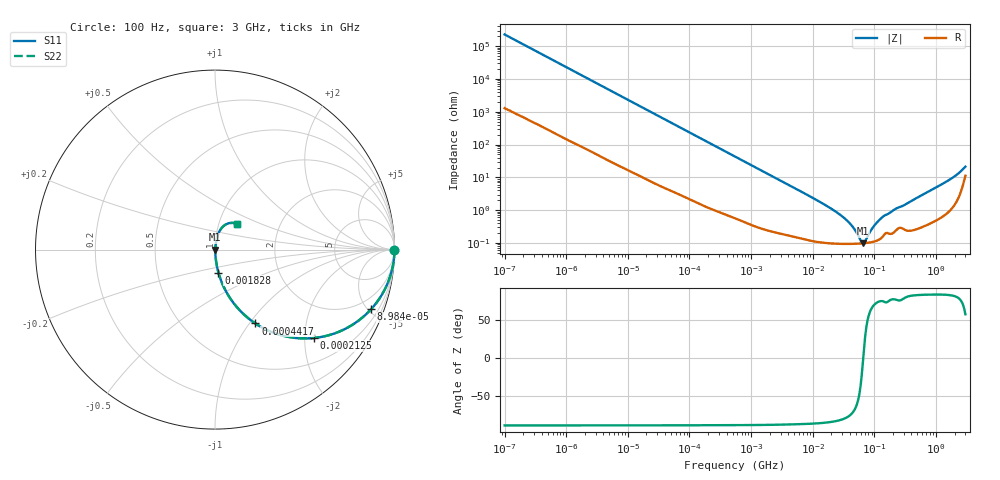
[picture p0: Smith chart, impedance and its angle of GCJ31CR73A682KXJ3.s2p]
!Murata Part Number: GCJ31CR73A682KXJ3
!These Parameters are Measured in Series Mode Connection
!Data Generated on Mar 13, 2026
!  o--ll--o
!Port1  Port2
!  o------o
!Operation Temp=25[degC], DC Bias Voltage=0[V]
!Freq. Start=100[Hz] Stop=3[GHz] 401[Steps]
# Hz S RI R 50
!Freq.(Hz) S11(Real) S11(Imag) S21(Real) S21(Imag) S12(Real) S12(Imag) S22(Real) S22(Imag)
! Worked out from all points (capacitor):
!   401 points, 100 Hz to 3 GHz, reference 50 ohm
!   read as one part in series: C = 7 nF near 109 Hz
!   lowest |Z| = 98.1 mohm at 65.08 MHz (marker M1)
!   series resonance near 65.93 MHz, so ESL is about 830 pH
!   S11 on the Smith chart (normalised r, x): 100 Hz: open; 89.84 kHz: 1.05, -5.21; 212.5 kHz: 1.02, -2.21; 441.7 kHz: 1.01, -1.07; 1.828 MHz: 1.00, -0.26; 3 GHz: 1.22, +0.36
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100  1 -0.00044  2.7e-06 0.00044  2.7e-06 0.00044  1 -0.00044
1788  0.9999 -0.00778  0.000112 0.00778  0.000112 0.00778  0.9999 -0.00778
10443  0.9976 -0.045  0.00236 0.045  0.00236 0.045  0.9976 -0.045
31977  0.9804 -0.1346  0.0196 0.1346  0.0196 0.1346  0.9804 -0.1346
89839  0.8692 -0.3327  0.1308 0.3327  0.1308 0.3327  0.8692 -0.3327
212480  0.5496 -0.4924  0.4504 0.4924  0.4504 0.4924  0.5496 -0.4924
441669  0.2251 -0.4114  0.7749 0.4114  0.7749 0.4114  0.2251 -0.4114
547723  0.1604 -0.3604  0.8396 0.3604  0.8396 0.3604  0.1604 -0.3604
918067  0.0658 -0.2406  0.9342 0.2406  0.9342 0.2406  0.0658 -0.2406
1827928  0.019 -0.1276  0.981 0.1276  0.981 0.1276  0.019 -0.1276
9794414  0.00173 -0.0241  0.9983 0.0241  0.9983 0.0241  0.00173 -0.0241
3.268714e7  0.000968 -0.00561  0.999 0.00561  0.999 0.00561  0.000968 -0.00561
4.418008e7  0.000949 -0.00304  0.9991 0.00304  0.9991 0.00304  0.000949 -0.00304
5.9714e7  0.000964 -0.000733  0.999 0.000733  0.999 0.000733  0.000964 -0.000733
6.508213e7  0.000976 -9.45e-05  0.999 9.45e-05  0.999 9.45e-05  0.000976 -9.45e-05
7.093284e7  0.000991 0.000545  0.999 -0.000545  0.999 -0.000545  0.000991 0.000545
8.79653e7  0.00105 0.00218  0.9989 -0.00218  0.9989 -0.00218  0.00105 0.00218
1.090876e8  0.00118 0.00395  0.9988 -0.00395  0.9988 -0.00395  0.00118 0.00395
1.352818e8  0.00156 0.00594  0.9984 -0.00594  0.9984 -0.00594  0.00156 0.00594
1.751444e8  0.00197 0.00789  0.998 -0.00789  0.998 -0.00789  0.00197 0.00789
1.71441e9  0.0173 0.0854  0.9827 -0.0854  0.9827 -0.0854  0.0173 0.0854
3e9  0.124 0.1421  0.876 -0.1421  0.876 -0.1421  0.124 0.1421
